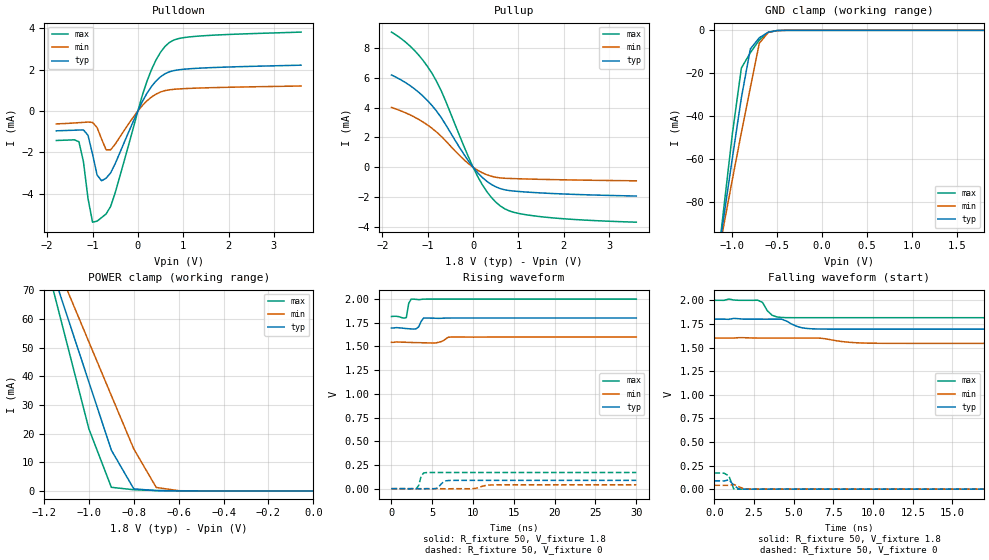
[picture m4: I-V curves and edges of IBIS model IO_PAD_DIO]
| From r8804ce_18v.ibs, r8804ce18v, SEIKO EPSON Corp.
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[Model]   IO_PAD_DIO
Model_type I/O
Enable Active-High
Polarity Non-Inverting
Vinh=1.6
Vinl=0.32
Vmeas=0.90
C_comp   2.5p   2.0p   3.0p
[Temperature Range] 25   105   -40
[Voltage Range]   1.8   1.6   2.0
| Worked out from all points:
|   slope of the pulldown table from 0 to 0.27 V, typ, clamps not added: 249 ohm
|   slope of the pullup table from 0 to 0.27 V, typ, clamps not added: 316 ohm
|   GND clamp passes 1 mA (typ) near -0.61 V on its own axis
|   POWER clamp passes 1 mA (typ) near -0.80 V on its own axis
|   falling waveform, R_fixture 50, V_fixture 1.8: 20-80 % time 809ps typ, 1.4ns min, 487ps max; typ from 1.8 V to 1.7 V
|   falling waveform, R_fixture 50, V_fixture 0: 20-80 % time 339ps typ, NA min, 224ps max; typ from 0.088 V to 0 V
|   rising waveform, R_fixture 50, V_fixture 1.8: 20-80 % time 379ps typ, 630ps min, 252ps max; typ from 1.7 V to 1.8 V
|   rising waveform, R_fixture 50, V_fixture 0: 20-80 % time 564ps typ, NA min, 352ps max; typ from 0 V to 0.088 V
[Pullup]
-1.8V     6.186mA    4.013mA    9.06mA
-1.3V     5.273mA    3.375mA    7.854mA
-1.1V     4.756mA    3.025mA    7.148mA
-900mV    4.116mA    2.598mA    6.265mA
-700mV    3.314mA    2.066mA    5.107mA
-200mV    857.2uA    503.2uA    1.393mA
100mV     -362uA     -200uA     -615.4uA
300mV     -933uA     -499.1uA   -1.618mA
600mV     -1.433mA   -714.2uA   -2.593mA
900mV     -1.596mA   -761.3uA   -3.022mA
1.4V      -1.705mA   -803.7uA   -3.28mA
3.6V      -1.929mA   -908.6uA   -3.682mA
[Pulldown]
-1.8V     -961.5uA   -625.3uA   -1.43mA
-1.3V     -922.8uA   -565.9uA   -1.492mA
-1.2V     -918.1uA   -552uA     -2.462mA
-1.1V     -1.178mA   -539uA     -4.238mA
-1V       -2.093mA   -553.4uA   -5.388mA
-900mV    -3.101mA   -801.9uA   -5.336mA
-700mV    -3.256mA   -1.879mA   -4.987mA
-600mV    -2.995mA   -1.879mA   -4.62mA
200mV     855.8uA    491.6uA    1.436mA
600mV     1.806mA    987.6uA    3.13mA
1.2V      2.053mA    1.099mA    3.601mA
3.6V      2.219mA    1.21mA     3.821mA
[GND Clamp]
-1.8V     -292.6mA   -252.9mA   -346.4mA
-1.2V     -117.3mA   -114.6mA   -121.6mA
-1.1V     -88.33mA   -91.95mA   -84.56mA
-1V       -59.57mA   -69.57mA   -48.26mA
-900mV    -31.49mA   -47.77mA   -17.61mA
-800mV    -8.683mA   -26.7mA    -10.45mA
-700mV    -3.453mA   -6.033mA   -4.512mA
-600mV    -868.8uA   -930.5uA   -956.3uA
-500mV    -86.23uA   -135.6uA   -52.66uA
-400mV    -4.725uA   -14.69uA   -1.074uA
1.8V      19.1pA     5.566nA    9.265pA
[POWER Clamp]
-1.8V     229.3mA    202.6mA    266.8mA
-1.2V     85.6mA     89.47mA    82.67mA
-1.1V     61.75mA    70.7mA     52.12mA
-1V       37.96mA    51.97mA    21.63mA
-900mV    14.22mA    33.28mA    1.266mA
-800mV    725.6uA    14.64mA    407.5uA
-700mV    111.9uA    1.216mA    132.2uA
-600mV    21.56uA    73.28uA    21.07uA
0V        19.1pA     599.4pA    11.94pA
[Falling Waveform]
R_fixture=50
V_fixture=1.8
V_fixture_min=1.6
V_fixture_max=2.0
0s        1.8V       1.6V       2V
2.727ns   1.8V       1.6V       2.001V
3.03ns    1.8V       1.6V       1.977V
3.333ns   1.8V       1.6V       1.889V
3.636ns   1.8V       1.6V       1.841V
4.242ns   1.8V       1.6V       1.818V
5.455ns   1.711V     1.6V       1.816V
6.364ns   1.697V     1.6V       1.816V
9.697ns   1.695V     1.546V     1.816V
30ns      1.695V     1.544V     1.816V
[Falling Waveform]
R_fixture=50
V_fixture=0
V_fixture_min=0
V_fixture_max=0
0s        87.71mV    40.74mV    170.6mV
606.1ps   86.11mV    40.09mV    168.5mV
909.1ps   99.07mV    40.36mV    141.6mV
1.212ns   42.58mV    50.36mV    2.808mV
1.515ns   2.834mV    28.27mV    68.71uV
1.818ns   412.2uV    5.199mV    2.323uV
2.121ns   46.18uV    1.624mV    -16.41uV
2.727ns   -9.488uV   197.4uV    1.284mV
3.03ns    -31.6uV    50.32uV    2.536mV
30ns      0V         0V         0V
[Rising Waveform]
R_fixture=50
V_fixture=1.8
V_fixture_min=1.6
V_fixture_max=2.0
0s        1.695V     1.544V     1.816V
1.818ns   1.689V     1.544V     1.805V
2.121ns   1.687V     1.543V     1.957V
2.424ns   1.685V     1.542V     2V
3.03ns    1.687V     1.541V     1.997V
3.333ns   1.707V     1.54V      1.994V
3.939ns   1.8V       1.539V     1.999V
5.455ns   1.798V     1.537V     2V
7.273ns   1.8V       1.599V     2V
30ns      1.8V       1.6V       2V
[Rising Waveform]
R_fixture=50
V_fixture=0
V_fixture_min=0
V_fixture_max=0
0s        0V         0V         0V
3.03ns    -128.6uV   23.12uV    -1.633mV
3.333ns   -760.3uV   28.23uV    34.13mV
3.636ns   -2.497mV   24.57uV    130.9mV
4.242ns   12.87uV    23.54uV    169.5mV
5.455ns   1.226mV    -14.49uV   170.5mV
6.97ns    86.14mV    -1.502mV   170.6mV
10ns      87.68mV    638uV      170.6mV
12.42ns   87.7mV     39.65mV    170.6mV
30ns      87.71mV    40.74mV    170.6mV
[Ramp]
R_load=50
dV/dt_r   5.262E-2/5.511E-10   2.445E-2/9.455E-10   1.024E-1/3.292E-10
dV/dt_f   6.318E-2/7.870E-10   3.371E-2/1.395E-9   1.106E-1/4.625E-10
|[End   IO_PAD_DIO
